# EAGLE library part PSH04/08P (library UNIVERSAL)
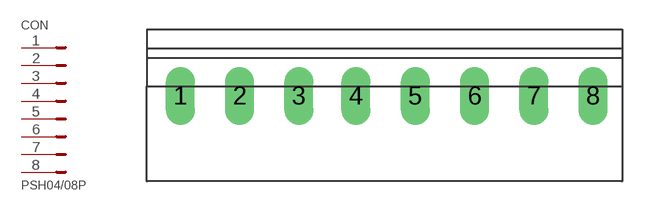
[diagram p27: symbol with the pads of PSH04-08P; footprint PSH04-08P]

Designator prefix CON

## PSH04/08P  [PSH04-08P]
1  1
2  2
3  3
4  4
5  5
6  6
7  7
8  8

## Footprint PSH04-08P (pad centres in mm)
drill 0.8 pad 1.93 long: 1 -7.93,0; 2 -3.97,0; 3 -0.01,0; 4 3.81,0; 5 7.77,0; 6 11.73,0; 7 15.69,0; 8 19.65,0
